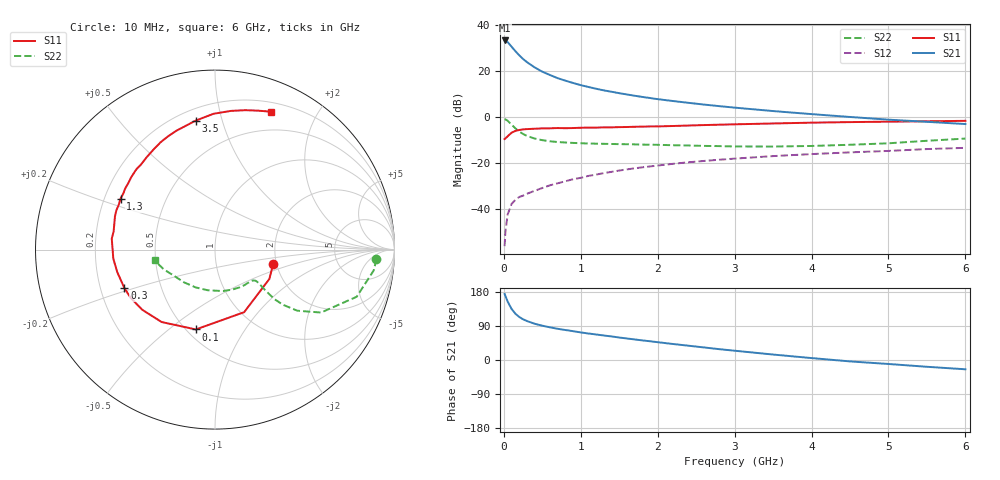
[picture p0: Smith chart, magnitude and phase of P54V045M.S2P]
! SIEMENS Small Signal Semiconductors
! BFP183
! Si NPN RF Bipolar Junction Transistor in SOT143
! VCE = 4 V  IC = 45 mA
! Common Emitter S-Parameters:  March  1996
# GHz  S  MA  R  50
!  f  S11  S21  S12  S22
! GHz  MAG  ANG  MAG  ANG  MAG  ANG  MAG  ANG
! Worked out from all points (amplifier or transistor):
!   36 points, 10 MHz to 6 GHz, reference 50 ohm
!   highest |S21| = 33.2 dB at 10 MHz (marker M1)
!   |S21| within 3 dB of that: start of sweep to 108.1 MHz
!   unconditionally stable (mu >= 1): start of sweep to 12.16 MHz; 441.1 MHz to end of sweep
!   at 250 MHz: K = 0.75, MSG = 29.6 dB, |S12| = -34.0 dB
!   at 1.4 GHz: K = 1.27, MAG = 14.2 dB, |S12| = -23.7 dB
!   at 6 GHz: K = 1.01, MAG = 4.6 dB, |S12| = -13.3 dB
!   S11 on the Smith chart (normalised r, x): 10 MHz: 1.92, -0.35; 100 MHz: 0.56, -0.63; 300 MHz: 0.30, -0.19; 1.3 GHz: 0.27, +0.24; 3.5 GHz: 0.27, +0.82; 6 GHz: 0.29, +1.44
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0.01  0.334 -14.1  45.62 174.4  0.0016 72.9  0.9012 -3.4
0.02  0.3442 -28.4  45.28 169.3  0.0033 75.9  0.8917 -7.5
0.05  0.3846 -65.0  41.97 153.9  0.0078 71.1  0.8321 -18.4
0.1  0.4575 -103.5  33.49 134.9  0.0131 57.9  0.6871 -30.7
0.15  0.5013 -126.4  26.78 122.2  0.0161 52.7  0.5708 -36.6
0.2  0.5257 -140.3  21.76 113.6  0.0186 51.7  0.4867 -39.1
0.25  0.5412 -150.0  18.1 107.4  0.0199 52.2  0.4311 -39.8
0.3  0.5485 -157.0  15.51 102.9  0.0218 52.8  0.3911 -39.4
0.4  0.5589 -167.1  11.93 95.7  0.0253 54.0  0.3429 -38.6
0.5  0.5688 -174.9  9.608 90.5  0.0291 55.0  0.3159 -37.8
0.6  0.571 179.3  8.136 86.2  0.0333 57.9  0.2988 -37.4
0.7  0.5785 173.9  6.957 82.4  0.0368 59.3  0.2881 -37.4
0.8  0.5738 169.9  6.143 79.1  0.0407 59.4  0.2814 -37.8
1.1  0.5916 158.2  4.484 69.9  0.0532 60.0  0.2677 -40.7
1.3  0.5978 151.7  3.784 64.6  0.0612 59.3  0.2634 -43.8
1.7  0.6164 139.4  2.897 54.3  0.0777 57.2  0.2563 -51.2
2.2  0.6407 126.3  2.225 42.2  0.0972 52.7  0.2454 -62.3
2.8  0.6837 112.3  1.725 28.6  0.1193 47.0  0.2351 -78.6
3.5  0.7267 98.5  1.349 14.4  0.1428 40.6  0.2301 -100.4
4.5  0.778 83.4  1.005 -3.7  0.1719 30.8  0.2513 -133.6
5.5  0.8104 72.8  0.789 -17.9  0.2028 22.4  0.3066 -159.1
6  0.8288 68.0  0.706 -24.5  0.2155 17.6  0.3422 -169.9
